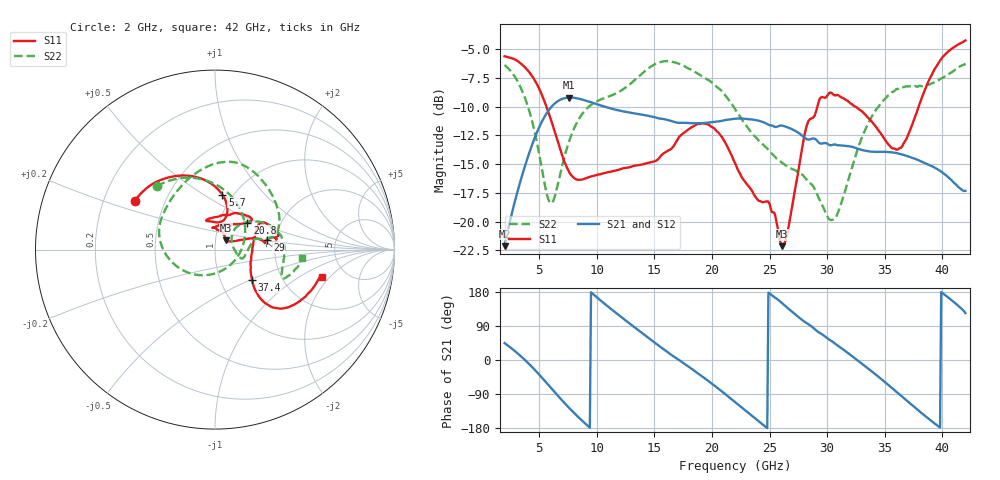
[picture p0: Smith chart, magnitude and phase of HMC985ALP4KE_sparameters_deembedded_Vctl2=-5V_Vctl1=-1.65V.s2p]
!s2p File: Measurements: S11, S21, S12, S22
# GHz S dB R 50.0
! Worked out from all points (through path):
!   401 points, 2 GHz to 42 GHz, reference 50 ohm
!   highest |S21| = -9.22 dB at 7.6 GHz (marker M1); lowest = -22.1 dB at 2 GHz (marker M2)
!   lowest |S11| = -22.1 dB at 26.1 GHz (marker M3), VSWR 1.17, Z = 56 + j5.72 ohm
!   |S11| at or under -10 dB: 5.631 GHz to 29.15 GHz (23.52 GHz wide, 135 % of centre); 32.42 GHz to 37.94 GHz (5.524 GHz wide, 15.7 % of centre)
!   |S22| runs from -19.9 to -6.0 dB; largest |S21 - S12| = 0.00035
!   S11 on the Smith chart (normalised r, x): 2 GHz: 0.33, +0.25; 5.7 GHz: 0.89, +0.60; 20.8 GHz: 1.36, +0.44; 29 GHz: 1.81, +0.22; 37.4 GHz: 1.41, -0.51; 42 GHz: 3.31, -1.62
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2  -5.62 148.7  -22.11 44.5  -22.11 44.5  -6.39 132.6
3.6  -6.43 122.3  -15.71 4.8  -15.71 4.8  -8.83 89.0
4.7  -7.86 101.3  -12.50 -28.5  -12.50 -28.5  -12.60 46.9
5.7  -10.19 82.4  -10.50 -62.3  -10.51 -62.3  -17.74 -20.6
6.3  -12.02 74.4  -9.78 -83.2  -9.78 -83.2  -17.99 -78.8
7.6  -15.68 75.3  -9.22 -126.4  -9.22 -126.4  -13.01 -152.4
8.7  -16.35 88.9  -9.38 -159.3  -9.38 -159.3  -10.69 178.6
12.1  -15.43 106.8  -10.38 114.0  -10.38 114.0  -8.61 131.7
15.4  -14.49 82.2  -11.03 37.5  -11.03 37.5  -6.18 83.8
18  -11.95 50.3  -11.43 -18.3  -11.44 -18.3  -6.70 53.8
20.8  -12.56 39.9  -11.25 -81.4  -11.25 -81.4  -8.60 18.4
22  -14.90 52.0  -11.05 -111.0  -11.06 -111.0  -10.21 12.1
24  -18.14 92.0  -11.21 -160.3  -11.22 -160.3  -12.89 14.3
26.1  -22.13 40.4  -11.65 149.6  -11.66 149.6  -14.89 -3.0
28.7  -11.00 7.4  -12.79 87.4  -12.79 87.4  -16.81 -17.3
29  -10.55 10.8  -12.84 79.3  -12.84 79.3  -17.31 -16.0
30.7  -9.03 14.7  -13.30 42.9  -13.30 43.0  -19.72 25.3
33.2  -10.60 30.3  -13.81 -14.1  -13.82 -14.1  -12.26 39.7
35.4  -13.36 7.9  -13.95 -68.1  -13.96 -68.1  -8.97 18.2
37.4  -11.53 -39.0  -14.46 -119.8  -14.46 -119.7  -8.27 -3.4
39.7  -6.14 -41.8  -15.52 -176.1  -15.52 -176.1  -7.69 -23.0
42  -4.25 -14.4  -17.32 123.9  -17.32 123.9  -6.25 -5.6
